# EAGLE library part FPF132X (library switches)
Digital Power Switch to select between two supply voltages 1.5-5.5V, 1.5A X=0/1 chooses whether Vout floats or is grounded when EN is low
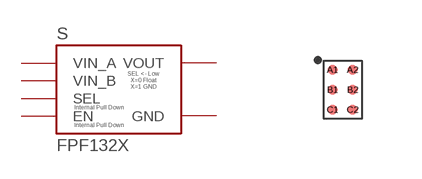
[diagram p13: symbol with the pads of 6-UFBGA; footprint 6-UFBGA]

Designator prefix S

## FPF132X-X=0 (DIGIKEY: FPF1320UCXCT-ND; MANUFACTURER: Fairchild/ON Semiconductor; MPN: FPF1320UCX)  [6-UFBGA]
A1  EN
A2  VIN_A
B1  SEL
B2  VOUT
C1  GND
C2  VIN_B

## FPF132X-X=1 (DIGIKEY: FPF1321UCXTR-ND; MANUFACTURER: Fairchild/ON Semiconductor; MPN: FPF1321UCX)  [6-UFBGA]
Pads as for 6-UFBGA

## Footprint 6-UFBGA (pad centres in mm)
6-Ball, 1.0 x 1.5 mm , Wafter-Level Chip-Scale Package (WLCSP) Drawn from https://www.fairchildsemi.com/datasheets/FP/FPF1321.pdf Digi-Key FPF1320UCXCT-ND
smd 0.25 x 0.25: A1 -0.25,0.5; A2 0.25,0.5; B1 -0.25,0; B2 0.25,0; C1 -0.25,-0.5; C2 0.25,-0.5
